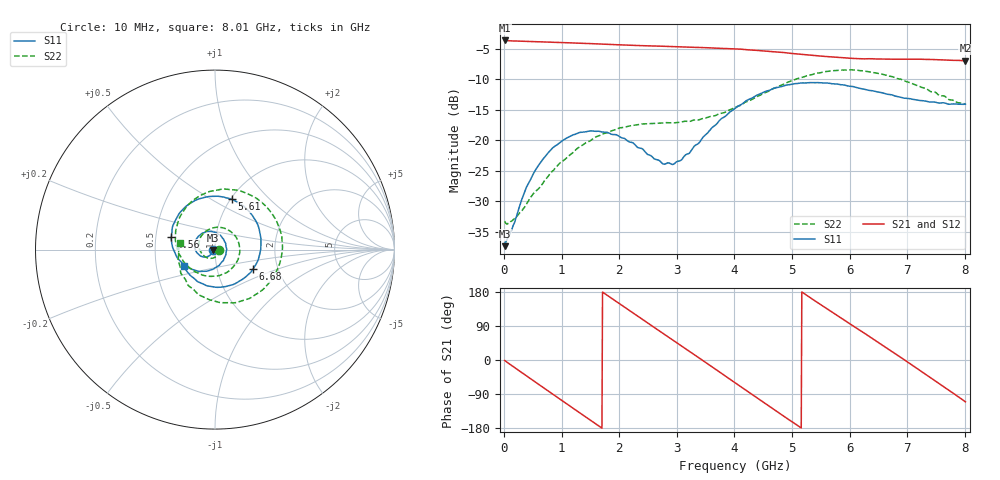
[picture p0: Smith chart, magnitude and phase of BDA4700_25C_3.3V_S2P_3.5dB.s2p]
!Agilent Technologies,E5071B,MY42404982,A.09.10
!Date: Mon Oct 20 18:04:27 2025
!Data & Calibration Information:
!Freq	S11:SOLT2(ON)	S21:SOLT2(ON)	S12:SOLT2(ON)	S22:SOLT2(ON)
# Hz S RI R 50
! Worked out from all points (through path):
!   801 points, 10 MHz to 8.01 GHz, reference 50 ohm
!   highest |S21| = -3.61 dB at 10 MHz (marker M1); lowest = -6.9 dB at 8.01 GHz (marker M2)
!   group delay of S21, straight-line fit = 287 ps
!   lowest |S11| = -37.3 dB at 10 MHz (marker M3), VSWR 1.03, Z = 48.7 - j0.151 ohm
!   |S11| at or under -10 dB: start of sweep to end of sweep
!   |S22| runs from -33.7 to -8.4 dB; largest |S21 - S12| = 0.0074
!   S11 on the Smith chart (normalised r, x): 10 MHz: 0.97, -0.00; 4.56 GHz: 0.60, +0.09; 5.61 GHz: 1.01, +0.62; 6.68 GHz: 1.49, -0.34; 8.01 GHz: 0.69, -0.13
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1e7  -0.0135 -0.00155  0.6595 -0.014  0.6594 -0.0148  0.0217 -0.00183
3.3e8  -0.0227 -0.0266  0.5287 -0.3773  0.5284 -0.3778  0.0195 -0.0191
7.2e8  -0.0621 -0.041  0.1458 -0.6239  0.1459 -0.6237  -0.00951 -0.0469
1.02e9  -0.0977 -0.0209  -0.2001 -0.6009  -0.2003 -0.601  -0.0545 -0.0403
1.35e9  -0.1135 0.0271  -0.5003 -0.3752  -0.5003 -0.3752  -0.0892 0.0153
1.64e9  -0.0943 0.0725  -0.6132 -0.0701  -0.6136 -0.07  -0.0725 0.0809
1.93e9  -0.0506 0.0994  -0.5578 0.2456  -0.5578 0.2458  -0.00595 0.1221
2.32e9  0.0173 0.0857  -0.2611 0.5398  -0.2607 0.5402  0.0988 0.0912
2.68e9  0.0589 0.0356  0.118 0.5808  0.117 0.5804  0.1383 -0.0106
3.06e9  0.0556 -0.0395  0.4548 0.3674  0.4508 0.3709  0.0858 -0.1117
3.36e9  0.016 -0.0919  0.5725 0.0811  0.5732 0.081  0.0041 -0.1467
3.67e9  -0.0577 -0.1203  0.5207 -0.2341  0.5207 -0.2356  -0.0883 -0.1334
4.01e9  -0.1551 -0.0968  0.2825 -0.4861  0.2833 -0.4852  -0.1722 -0.0704
4.56e9  -0.2436 0.0706  -0.2481 -0.4785  -0.2475 -0.4791  -0.2134 0.128
4.97e9  -0.1773 0.2259  -0.4864 -0.1774  -0.4869 -0.1794  -0.1057 0.2863
5.35e9  -0.0253 0.2961  -0.4719 0.1619  -0.4726 0.1594  0.0935 0.3334
5.61e9  0.0936 0.2802  -0.3433 0.3446  -0.3436 0.3448  0.2358 0.2821
6.12e9  0.2446 0.1172  0.0494 0.4661  0.0524 0.4669  0.3761 0.0163
6.68e9  0.2119 -0.1088  0.4101 0.2161  0.4112 0.2155  0.2215 -0.2541
7.24e9  0.0338 -0.2092  0.4025 -0.2284  0.4017 -0.2288  -0.0576 -0.2671
7.63e9  -0.0941 -0.1804  0.1534 -0.4294  0.153 -0.4301  -0.1887 -0.1347
8.01e9  -0.1748 -0.0934  -0.1562 -0.4215  -0.1549 -0.4221  -0.1957 0.037
